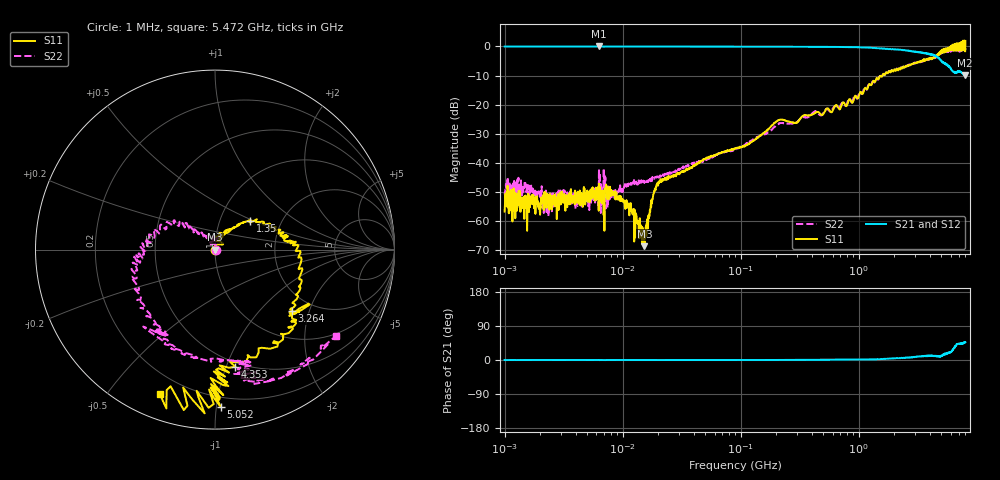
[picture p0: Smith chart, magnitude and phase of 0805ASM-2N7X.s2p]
!s-Parameter Generated by FASTRON Sdn. Bhd.
!FASTRON P/N : 0805ASM-2N7X
!Keysight Technologies: E5071C_MY46733604_B.14.02
!Date: Fri Jun 19 14:46:02 2026
!Version  :Rev00  Fri Jun 19 14:46:02 2026
!Data & Calibration Information:
!Freq  S11:SOLT2(ON)  S21:SOLT2(ON)  S12:SOLT2(ON)  S22:SOLT2(ON)
!PortZ  Port1:50+j0  Port2:50+j0
!When reading reference impedance value at option line is always used.
! Remarks : This data is being provided solely for informational purposes.
# Hz S dB R 50
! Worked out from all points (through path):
!   1601 points, 1 MHz to 8 GHz, reference 50 ohm
!   highest |S21| = 0.01 dB at 6.301 MHz (marker M1); lowest = -9.9 dB at 7.923 GHz (marker M2)
!   lowest |S11| = -68.6 dB at 15.27 MHz (marker M3), VSWR 1.00, Z = 50 - j0.0204 ohm
!   |S11| at or under -10 dB: start of sweep to 1.588 GHz
!   |S22| runs from -58.4 to -0.4 dB; largest |S21 - S12| = 0.0095
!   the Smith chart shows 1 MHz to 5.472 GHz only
!   S11 on the Smith chart (normalised r, x): 1 MHz: 1.00, -0.00; 1.35 GHz: 1.39, +0.47; 3.264 GHz: 1.59, -1.54; 4.353 GHz: 0.46, -1.08; 5.052 GHz: 0.13, -1.03; 5.472 GHz: 0.11, -0.68
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1000000  -56.70 -48.6  -0.03 -0.1  -0.03 -0.1  -50.30 -6.9
1550103  -63.30 -55.9  -0.03 -0.1  -0.02 -0.1  -48.60 -30.8
2248791  -54.00 -0.7  -0.03 -0.1  -0.04 -0.1  -53.20 1.3
4479405  -52.50 1.4  -0.03 -0.0  -0.03 -0.1  -53.00 13.0
6301378  -47.10 21.3  0.01 -0.2  -0.01 -0.2  -42.00 35.8
1.120536e7  -54.70 1.3  -0.03 -0.1  -0.04 -0.1  -47.10 24.7
1.526847e7  -68.60 -33.3  -0.02 -0.1  -0.04 -0.1  -46.90 28.8
2.00676e7  -46.80 42.2  -0.03 -0.1  -0.05 -0.0  -44.90 54.1
8.994653e7  -35.00 75.7  -0.05 -0.1  -0.06 -0.1  -35.30 71.9
2.089357e8  -25.30 33.7  -0.08 0.1  -0.10 0.1  -26.50 138.0
4.006501e8  -23.50 100.0  -0.12 0.4  -0.13 0.4  -23.10 78.1
1.349549e9  -12.00 39.1  -0.49 1.9  -0.50 1.8  -12.40 147.0
1.7949e9  -8.60 17.4  -0.93 3.5  -0.94 3.3  -8.47 167.0
3.26428e9  -5.22 -38.4  -2.06 10.0  -2.08 10.2  -5.21 -126.0
3.730463e9  -4.68 -43.3  -2.46 10.2  -2.47 10.4  -4.55 -116.0
4.352635e9  -3.58 -80.1  -3.03 11.3  -3.02 11.2  -4.04 -81.5
5.052431e9  -1.13 -87.9  -5.03 11.8  -5.01 11.3  -2.16 -73.7
5.472309e9  -1.30 -111.0  -6.10 15.0  -6.05 15.1  -1.63 -35.3
6.457806e9  -0.36 -121.0  -8.95 31.2  -8.85 31.1  -0.90 8.8
6.959019e9  -1.04 -140.0  -8.71 42.6  -8.65 41.9  -1.15 50.9
7.92289e9  1.25 -160.0  -9.87 46.8  -9.62 46.5  -0.38 83.9
8e9  1.90 -174.0  -9.59 47.0  -9.46 46.7  -0.57 81.4
